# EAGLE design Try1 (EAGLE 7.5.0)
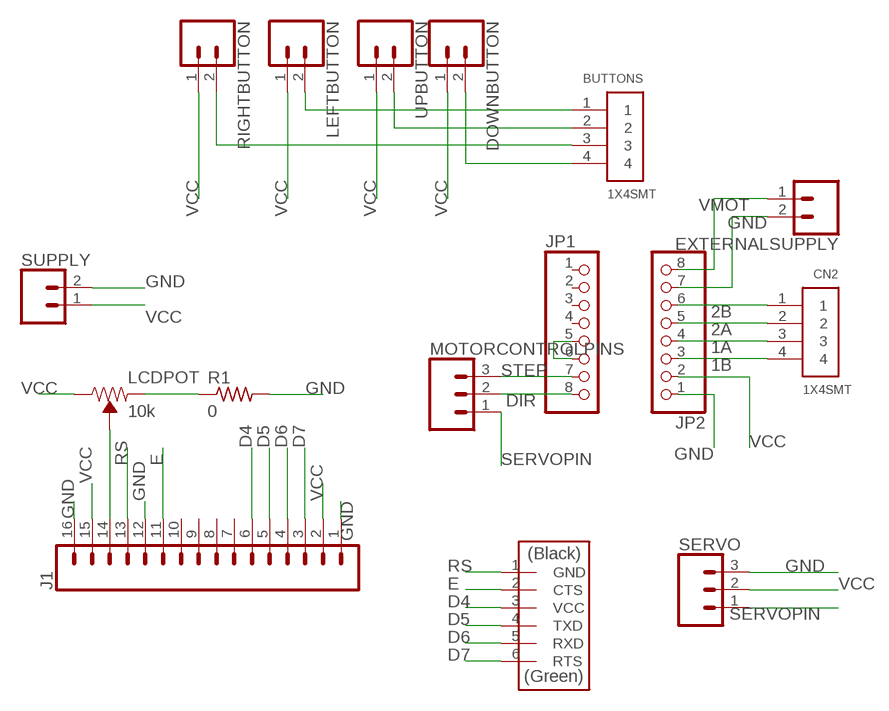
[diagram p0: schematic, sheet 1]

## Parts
BUTTONS  1X4SMT  [1X4-SMT]
CN2  1X4SMT  [1X4-SMT]
DOWNBUTTON  CONN_02  [1X02]
EXTERNALSUPPLY  CONN_02  [1X02]
J1  CONN_16LONGPADS  [1X16_LONGPADS]
JP1  PINHD-1X8CLEANBIG  [1X08-CLEANBIG]
JP2  PINHD-1X8CLEANBIG  [1X08-CLEANBIG]
LCDPOT  10k  TRIMPOT-PTH-10MM-KNOB-1/2W-10%  [TRIMPOT-PTH-3386U]
LEFTBUTTON  CONN_02  [1X02]
MOTORCONTROLPINS  CONN_03  [1X03]
R1  0  RES-US1206FAB  [R1206FAB]
RIGHTBUTTON  CONN_02  [1X02]
SERVO  CONN_03  [1X03]
SUPPLY  CONN_02  [1X02]
U$2  FTDI-SMD-HEADER  [1X06SMD]
UPBUTTON  CONN_02  [1X02]

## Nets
1A: CN2.3 JP2.4
1B: CN2.4 JP2.3
2A: CN2.2 JP2.5
2B: CN2.1 JP2.6
D4: J1.6 U$2.3(VCC)
D5: J1.5 U$2.4(TXD)
D6: J1.4 U$2.5(RXD)
D7: J1.3 U$2.6(RTS)
DIR: JP1.8 MOTORCONTROLPINS.2
E: J1.11 U$2.2(CTS)
GND: EXTERNALSUPPLY.2 J1.1 J1.12 J1.16 JP2.1 JP2.7 R1.2 SERVO.3 SUPPLY.2
N$1: BUTTONS.1 LEFTBUTTON.2
N$2: BUTTONS.3 RIGHTBUTTON.2
N$3: BUTTONS.2 UPBUTTON.2
N$4: BUTTONS.4 DOWNBUTTON.2
N$5: J1.14 LCDPOT.2(WIPER)
N$6: LCDPOT.1(CCW) R1.1
N$12: JP1.5 JP1.6
RS: J1.13 U$2.1(GND)
SERVOPIN: MOTORCONTROLPINS.1 SERVO.1
STEP: JP1.7 MOTORCONTROLPINS.3
VCC: DOWNBUTTON.1 J1.2 J1.15 JP2.2 LCDPOT.3(CW) LEFTBUTTON.1 RIGHTBUTTON.1 SERVO.2 SUPPLY.1 UPBUTTON.1
VMOT: EXTERNALSUPPLY.1 JP2.8
Unconnected: J1.7 J1.8 J1.9 J1.10 JP1.1 JP1.2 JP1.3 JP1.4

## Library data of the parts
BUTTONS CN2 = adafruit:1X4: 4-pin connector
DOWNBUTTON EXTERNALSUPPLY LEFTBUTTON RIGHTBUTTON SUPPLY UPBUTTON = SparkFun-Connectors:CONN_02: Multi connection point. Often used as Generic Header-pin footprint for 0.1 inch spaced/style header connections
J1 = SparkFun-Connectors:CONN_16: Multi connection point. Often used as Generic Header-pin footprint for 0.1 inch spaced/style header connections On any of the 0.1 inch spaced packages, you can populate with these: Break Away Headers - Straight (PRT-00116) Break Away Male Headers - Right Angle (PRT-00553) Female Headers (PRT-00115)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
JP1 JP2 = adafruit:PINHD-1X8: PIN HEADER
LCDPOT = SparkFun-Resistors:TRIMPOT: Trimming Potentiometer (Trimpot) Three-terminal potentiometers, with an adjustable wiper and two adjustable resistors. A pot can be used to create a configurable voltage divider, or as a variable resistor. "Trimpots" are a subset of potentiometers, usually intended for "set-and-forget"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; PROD_ID: RES-09730; SF_SKU: COM-09806
MOTORCONTROLPINS SERVO = SparkFun-Connectors:CONN_03: Multi connection point. Often used as Generic Header-pin footprint for 0.1 inch spaced/style header connections On any of the 0.1 inch spaced packages, you can populate with these: Break Away Headers - Straight (PRT-00116) Break Away Male Headers - Right Angle (PRT-00553) Female Headers (PRT-00115)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
R1 = fab:RES-US: Resistor (US Symbol)
U$2 = fab:FTDI-SMD-HEADER

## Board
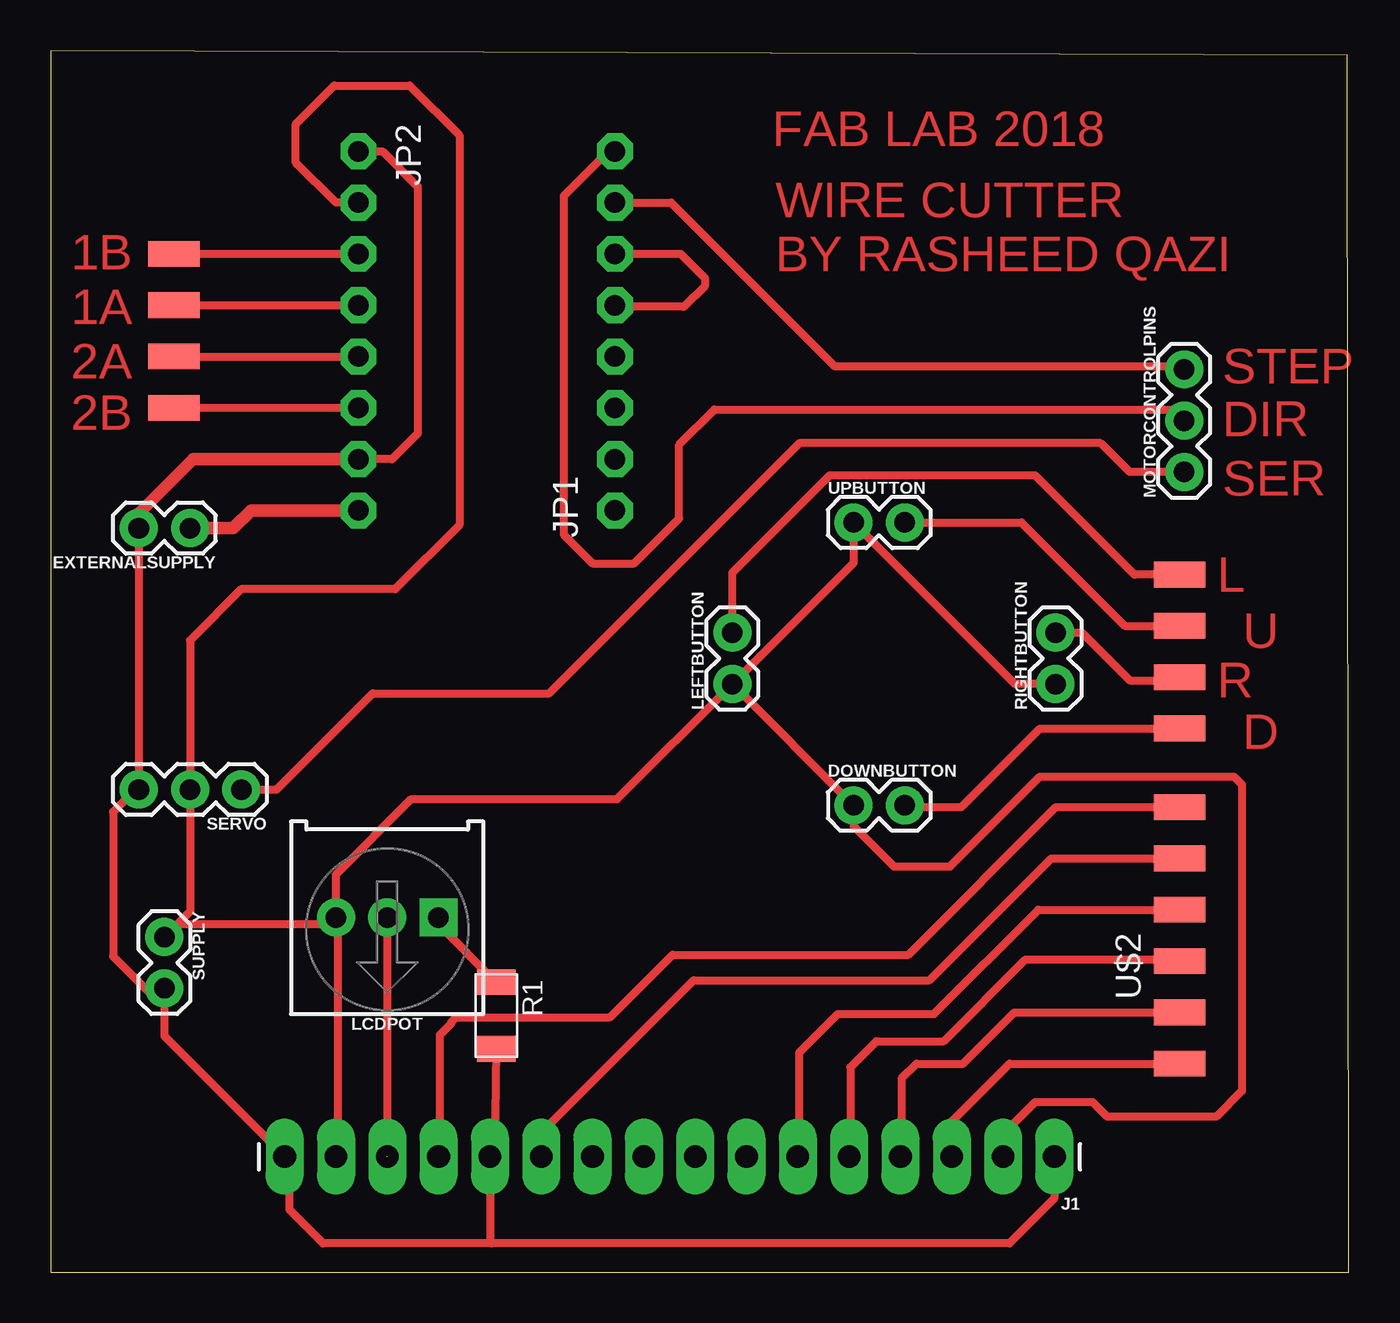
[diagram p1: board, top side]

Size 64.27 x 60.47 mm. Coordinates in mm from the lower left corner, seen from the top.
Outline: 0,0 64.27,0 64.19,60.23 0,60.47 0,0
Copper layers (1*16): Top 0.035mm / dielectric 1.5mm / Bottom 0.035mm
Design rules "default": minimum track width 10mil, minimum drill 24mil, track to track 8mil, track to pad 8mil, pad to pad 8mil, via to via 8mil, smd to smd 8mil, copper to edge 40mil, drill to drill 8mil, minimum pad ring 10mil, minimum via ring 8mil, stop-mask expansion 4mil, vias tented up to drill 0mil, thermal gap 10mil

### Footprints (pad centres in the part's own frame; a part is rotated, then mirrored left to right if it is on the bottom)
1X4-SMT = smd 1.27 x 2.54: 1 -3.81,0; 2 -1.27,0; 3 1.27,0; 4 3.81,0
1X02 = drill 1.016 pad 1.88: 1 0,0; 2 2.54,0
1X16_LONGPADS = drill 1.118 pad 1.88 long: 1 0,0; 2 2.54,0; 3 5.08,0; 4 7.62,0; 5 10.16,0; 6 12.7,0; 7 15.24,0; 8 17.78,0; 9 20.32,0; 10 22.86,0; 11 25.4,0; 12 27.94,0; 13 30.48,0; 14 33.02,0; 15 35.56,0; 16 38.1,0
1X08-CLEANBIG = drill 1.016 pad 1.778 octagon: 1 -8.89,0; 2 -6.35,0; 3 -3.81,0; 4 -1.27,0; 5 1.27,0; 6 3.81,0; 7 6.35,0; 8 8.89,0
TRIMPOT-PTH-3386U = drill 1.016 pad 1.88 square: 1 -2.54,-0.015 | drill 1.016 pad 1.88: 2 0,-0.015; 3 2.54,-0.015
1X03 = drill 1.016 pad 1.88: 1 0,0; 2 2.54,0; 3 5.08,0
R1206FAB = smd 1.27 x 1.905: 1 -1.651,0; 2 1.651,0
1X06SMD = smd 2.54 x 1.27: 1 0,6.35; 2 0,3.81; 3 0,1.27; 4 0,-1.27; 5 0,-3.81; 6 0,-6.35

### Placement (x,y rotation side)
BUTTONS  55.88,30.72 270 top
CN2  6.11,46.59 90 top
DOWNBUTTON  39.75,23.11 0 top
EXTERNALSUPPLY  6.91,36.83 180 top
J1  49.69,5.71 180 top
JP1  27.94,46.59 90 top
JP2  15.24,46.59 270 top
LCDPOT  16.67,17.54 180 top
LEFTBUTTON  33.75,29.11 90 top
MOTORCONTROLPINS  56.12,39.61 90 top
R1  22.07,12.7 270 top
RIGHTBUTTON  49.75,29.11 90 top
SERVO  9.45,23.89 180 top
SUPPLY  5.64,16.59 270 top
U$2  55.88,16.67 0 top
UPBUTTON  39.75,37.11 0 top

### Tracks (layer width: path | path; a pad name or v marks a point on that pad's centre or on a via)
1A
  Top 0.406: CN2.3 JP2.4
1B
  Top 0.406: CN2.4 JP2.3
2A
  Top 0.406: CN2.2 JP2.5
2B
  Top 0.406: CN2.1 JP2.6
D4
  Top 0.406: U$2.3 55.72,18.1 55.32,18.1 55.17,17.94 48.9,17.94 43.74,12.78 38.97,12.78 37.05,10.86 37.05,5.78 J1.6
D5
  Top 0.406: 55.8,15.48 U$2.4 56.04,15.24 56.44,15.24 56.2,15.48 48.26,15.48 44.21,11.43 40.88,11.43 39.59,10.14 39.59,6.13 40.08,5.64 40.08,5.4 39.85,5.4 J1.5
D6
  Top 0.406: U$2.5 47.7,12.86 45.16,10.32 42.86,10.32 42.13,9.59 42.13,5.78 J1.4
D7
  Top 0.406: U$2.6 47.47,10.32 44.67,7.52 44.67,5.78 J1.3
DIR
  Top 0.406: JP1.8 27.62,55.48 25.4,53.26 25.4,36.51 26.83,35.08 28.89,35.08 31.11,37.31 31.11,40.96 32.86,42.7 55.56,42.7 MOTORCONTROLPINS.2
E
  Top 0.406: U$2.2 49.53,20.48 43.5,14.45 31.83,14.45 24.29,6.91 J1.11
GND
  Top 0.406: JP2.1 16.43,55.48 18.18,53.74 18.18,41.51 16.91,40.24 JP2.7 | EXTERNALSUPPLY.2 SERVO.3 3.97,23.65 3.1,22.78 3.1,15.64 5.24,13.49 5.71,13.49 5.64,13.57 SUPPLY.2 5.64,11.69 11.59,5.74 J1.16 11.83,5.48 11.83,3.1 13.49,1.43 21.83,1.43 | R1.2 21.99,6.03 | 21.99,6.03 21.99,5.85 | 21.99,6.03 21.75,5.79 J1.12 21.75,1.51 21.83,1.43 | J1.1 49.69,3.65 47.47,1.43 21.83,1.43
  Top 0.61: JP2.7 7.06,40.24 4.37,37.54 EXTERNALSUPPLY.2
N$1
  Top 0.406: LEFTBUTTON.2 33.75,34.62 38.58,39.45 48.74,39.45 53.66,34.53 BUTTONS.1
N$2
  Top 0.406: RIGHTBUTTON.2 51.06,31.65 53.42,29.29 55.72,29.29 BUTTONS.3
N$3
  Top 0.406: UPBUTTON.2 48.06,37.11 53.18,31.99 BUTTONS.2
N$4
  Top 0.406: DOWNBUTTON.2 42.29,23.04 42.31,23.02 45.09,23.02 48.97,26.91 BUTTONS.4
N$5  (1 unrouted)
  Top 0.406: LCDPOT.2 16.67,5.74
N$6
  Top 0.406: LCDPOT.1 19.21,17.21 R1.1
N$12
  Top 0.406: JP1.6 31.19,50.4 32.38,49.21 32.38,48.82 31.35,47.78 28.81,47.78 JP1.5
RS
  Top 0.406: U$2.1 49.77,23.02 42.47,15.72 30.8,15.72 27.7,12.62 20.08,12.62 19.84,12.38 19.84,12.3 19.27,11.73 19.27,5.78 J1.13
SERVOPIN
  Top 0.406: MOTORCONTROLPINS.1 53.42,39.61 51.99,41.04 37.07,41.04 24.69,28.65 15.95,28.65 11.19,23.89 SERVO.1
STEP
  Top 0.406: JP1.7 30.72,52.94 38.81,44.85 55.96,44.85 MOTORCONTROLPINS.3
VCC
  Top 0.406: LEFTBUTTON.1 DOWNBUTTON.1 39.75,22.09 41.75,20.08 44.53,20.08 48.97,24.53 58.58,24.53 58.98,24.13 58.98,8.97 57.71,7.7 52.31,7.7 51.59,8.41 48.74,8.41 47.23,6.91 47.23,6.67 47.23,5.79 | LEFTBUTTON.1 39.75,35.11 UPBUTTON.1 47.75,29.11 RIGHTBUTTON.1 | LCDPOT.3 14.13,19.68 17.86,23.42 28.05,23.42 LEFTBUTTON.1 | 14.19,17.49 LCDPOT.3 | LCDPOT.3 14.13,17.3 14.21,17.22 | 14.21,17.22 6.27,17.22 SUPPLY.1 6.91,17.86 SERVO.2 6.91,31.27 9.45,33.81 17.07,33.81 20.24,36.99 20.24,56.28 17.78,58.74 14.05,58.74 12.14,56.83 12.14,54.93 14.13,52.94 JP2.2 | 14.21,17.22 14.21,5.79 J1.15 | 47.23,5.7 47.23,5.79 | 47.23,5.79 J1.2
VMOT
  Top 0.61: JP2.8 9.92,37.7 9.05,36.83 EXTERNALSUPPLY.1

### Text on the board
Top: FAB LAB 2018 | 1B | WIRE CUTTER / BY RASHEED QAZI | 1A | 2A | STEP | 2B | DIR | SER | L | U | R | D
